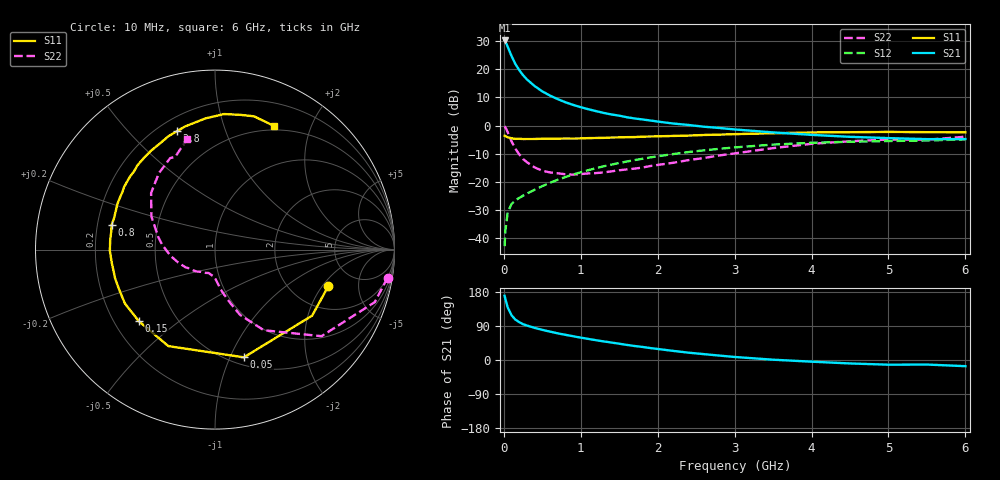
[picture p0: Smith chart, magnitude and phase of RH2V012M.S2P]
! SIEMENS Small Signal Semiconductors
! BFR106
! Si NPN RF Bipolar Junction Transistor in SOT23
! VCE = 2 V  IC = 12 mA
! Common Emitter S-Parameters:  August  1996
# GHz  S  MA  R  50
!  f  S11  S21  S12  S22
! GHz  MAG  ANG  MAG  ANG  MAG  ANG  MAG  ANG
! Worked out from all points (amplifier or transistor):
!   36 points, 10 MHz to 6 GHz, reference 50 ohm
!   highest |S21| = 30.2 dB at 10 MHz (marker M1)
!   |S21| within 3 dB of that: start of sweep to 62.01 MHz
!   unconditionally stable (mu >= 1): 437.3 MHz to 2.38 GHz; 4.788 GHz to end of sweep
!   at 250 MHz: K = 0.78, MSG = 21.4 dB, |S12| = -24.8 dB
!   at 1.4 GHz: K = 1.10, MAG = 7.0 dB, |S12| = -13.8 dB
!   at 6 GHz: K = 1.02, MAG = -0.8 dB, |S12| = -4.9 dB
!   S11 on the Smith chart (normalised r, x): 10 MHz: 3.17, -2.30; 50 MHz: 0.58, -1.13; 150 MHz: 0.30, -0.36; 800 MHz: 0.26, +0.11; 2.8 GHz: 0.27, +0.69; 6 GHz: 0.45, +1.49
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0.01  0.6636 -17.8  32.34 169.5  0.0073 83.5  0.9744 -9.2
0.02  0.6544 -34.2  30.98 161.0  0.0137 77.0  0.9372 -18.2
0.05  0.6213 -75.0  25.08 138.7  0.0289 59.6  0.7648 -39.1
0.1  0.5972 -115.8  17.14 118.1  0.0408 47.9  0.5252 -58.8
0.15  0.5824 -136.8  12.36 106.6  0.0474 45.5  0.3897 -69.0
0.2  0.5849 -149.1  9.672 99.9  0.0523 46.1  0.3099 -74.0
0.25  0.5785 -157.6  7.826 94.5  0.0573 47.5  0.255 -78.6
0.3  0.5792 -163.9  6.59 90.9  0.0624 50.0  0.2252 -81.7
0.4  0.5797 -172.8  5.025 84.8  0.0729 53.3  0.1819 -86.3
0.5  0.5857 -179.3  4.05 79.5  0.0847 56.2  0.1582 -90.2
0.6  0.5863 175.1  3.405 74.9  0.097 57.8  0.1482 -93.8
0.7  0.5868 170.2  2.95 70.4  0.1097 59.1  0.1428 -98.2
0.8  0.5922 166.5  2.595 66.5  0.1225 59.4  0.1374 -102.5
1.1  0.6006 154.8  1.949 55.5  0.1626 59.6  0.1424 -115.0
1.3  0.6068 148.4  1.679 49.0  0.1905 58.2  0.148 -123.6
1.6  0.6246 139.2  1.407 39.8  0.2314 55.6  0.1675 -136.5
2.2  0.6562 122.9  1.091 24.1  0.3133 48.1  0.2193 -161.5
2.8  0.6926 108.0  0.909 11.7  0.3879 38.8  0.2958 174.5
3.5  0.7325 94.3  0.758 0.8  0.4614 27.5  0.3995 152.5
4.5  0.764 79.3  0.633 -9.1  0.5176 11.6  0.5281 126.3
5.5  0.7653 68.3  0.576 -12.0  0.5448 1.8  0.562 113.2
6  0.7629 64.4  0.578 -16.3  0.5708 -5.4  0.6367 104.1
